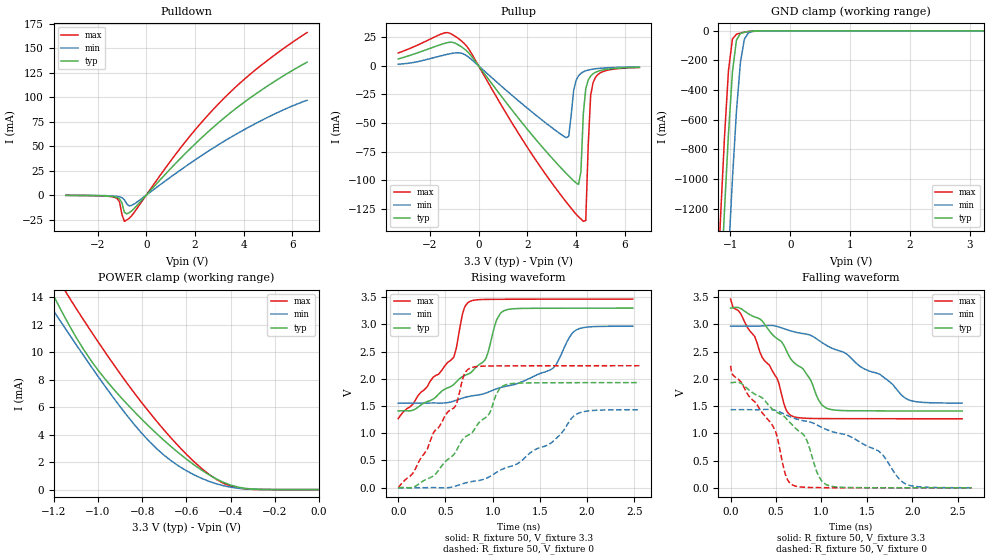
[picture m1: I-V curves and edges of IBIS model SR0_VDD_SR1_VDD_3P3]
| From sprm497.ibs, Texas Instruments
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|SR0_VSS_SR1_VSS_3P3CELL OPERATING IN SLOW MODE
|   Model Cell SR0_VDD_SR1_VDD_3P3
|SR0_VDD_SR1_VDD_3P3
[Model]   SR0_VDD_SR1_VDD_3P3
Model_type   I/O
Polarity   Non-Inverting
Enable   Active-Low
Vinl =  0.8V
Vinh =  2V
Cref =  5.0000pF
Rref =  100.0000M
Vref =  0V
Vmeas =  1.65
C_comp   2.088321p   2.017362p   2.221145p
[Model Spec]
Vinl   0.8V   0.8V   0.8V
Vinh   2V   2V   2V
[Temperature Range]   25   125   -40
[Voltage Range]   3.3   2.97   3.465
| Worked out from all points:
|   slope of the pulldown table from 0 to 0.495 V, typ, clamps not added: 36.4 ohm
|   slope of the pullup table from 0 to 0.495 V, typ, clamps not added: 34.9 ohm
|   GND clamp passes 1 mA (typ) near -0.57 V on its own axis
|   POWER clamp passes 1 mA (typ) near -0.49 V on its own axis
|   rising waveform, R_fixture 50, V_fixture 3.3: 20-80 % time 541ps typ, 710ps min, 445ps max; typ from 1.41 V to 3.3 V
|   rising waveform, R_fixture 50, V_fixture 0: 20-80 % time 550ps typ, 740ps min, 446ps max; typ from 0 V to 1.93 V
|   falling waveform, R_fixture 50, V_fixture 3.3: 20-80 % time 515ps typ, 823ps min, 401ps max; typ from 3.3 V to 1.41 V
|   falling waveform, R_fixture 50, V_fixture 0: 20-80 % time 525ps typ, 841ps min, 409ps max; typ from 1.93 V to 0.001 V
[POWER_clamp]
|   voltage   I(typ)   I(min)   I(max)
-3.3V     86.08mA    64.51mA    104.3mA
-1.267V   16.23mA    14.61mA    17.94mA
-1.233V   15.14mA    13.79mA    16.86mA
-1.2V     14.07mA    12.98mA    15.86mA
-1.133V   12.04mA    11.37mA    14.06mA
-1V       8.693mA    8.239mA    10.76mA
-866.7mV  6.192mA    5.342mA    7.695mA
-766.7mV  4.556mA    3.483mA    5.603mA
-633.3mV  2.644mA    1.698mA    3.12mA
-500mV    1.095mA    613.6uA    1.135mA
-366.7mV  181.9uA    101.9uA    111.5uA
-11.55fV  484.7nA    452.9nA    508.6nA
[Pulldown]
|   voltage   I(typ)   I(min)   I(max)
-3.3V     -240.7uA   -171.6uA   -267.5uA
-1.3V     -1.697mA   -968uA     -2.239mA
-1.1V     -3.762mA   -1.687mA   -6.636mA
-1V       -7.727mA   -2.567mA   -19.64mA
-900mV    -17.44mA   -4.637mA   -26.73mA
-800mV    -19.19mA   -8.992mA   -25.39mA
-700mV    -17.88mA   -11mA      -23.57mA
-500mV    -13.74mA   -9.146mA   -17.83mA
1.4V      37.42mA    25.57mA    48.03mA
2.9V      72.6mA     50.52mA    91.53mA
4.6V      105.1mA    74.64mA    130.4mA
6.6V      135.8mA    96.92mA    166.1mA
[Pullup]
|   voltage   I(typ)   I(min)   I(max)
-3.3V     6.015mA    1.488mA    11.26mA
-1.4V     19.63mA    9.503mA    28.79mA
-700mV    16.55mA    11.01mA    21.71mA
3.6V      -93.97mA   -62.77mA   -119mA
4.1V      -103.6mA   -8.736mA   -131.8mA
4.2V      -92.66mA   -6.55mA    -133.7mA
4.3V      -41.55mA   -5.211mA   -135.8mA
4.4V      -19.91mA   -4.314mA   -135.1mA
4.5V      -12.4mA    -3.675mA   -69.72mA
4.6V      -8.868mA   -3.197mA   -25.86mA
4.7V      -6.864mA   -2.828mA   -14.55mA
6.6V      -1.25mA    -873.6uA   -1.41mA
[GND_clamp]
|   voltage   I(typ)   I(min)   I(max)
-3.3V     -22.46A    -23.25A    -22.02A
-1.233V   -2.372A    -3.255A    -1.856A
-1.167V   -1.78A     -2.658A    -1.268A
-1.1V     -1.214A    -2.077A    -719.3mA
-1.033V   -694.8mA   -1.519A    -269mA
-966.7mV  -277.7mA   -998.2mA   -54.71mA
-900mV    -62.85mA   -543.8mA   -23.11mA
-833.3mV  -17.76mA   -212.7mA   -15.05mA
-766.7mV  -9.254mA   -55.4mA    -9.029mA
-700mV    -5.096mA   -13.88mA   -4.435mA
-633.3mV  -2.353mA   -4.844mA   -1.587mA
3.233V    464.9nA    13.45uA    453.9nA
[Ramp]
| variable   typ   min   max
dV/dt_f   1.523623/0.6823479n   1.142936/1.116097n   1.76944/0.5156569n
dV/dt_r   1.547097/0.6949547n   1.150652/0.9660429n   1.794801/0.5503525n
R_load = 50
[Rising Waveform]
R_fixture = 50
V_fixture = 3.3
V_fixture_min = 2.97
V_fixture_max = 3.465
|   time   V(typ)   V(min)   V(max)
0s        1.411V     1.554V     1.269V
588ps     1.894V     1.591V     2.394V
679ps     2.04V      1.645V     3.177V
749ps     2.094V     1.677V     3.413V
931ps     2.384V     1.74V      3.459V
1.043ns   3.086V     1.817V     3.461V
1.12ns    3.252V     1.856V     3.462V
1.638ns   3.297V     2.191V     3.464V
1.89ns    3.298V     2.902V     3.464V
2.485ns   3.299V     2.967V     3.465V
[Rising Waveform]
R_fixture = 50
V_fixture = 0
V_fixture_min = 0
V_fixture_max = 0
|   time   V(typ)   V(min)   V(max)
0s        5.618uV    6.879uV    4.844uV
154ps     4.714mV    -39.95uV   260.1mV
371ps     213.5mV    2.931mV    1.004V
616ps     679.6mV    34.54mV    1.524V
679ps     878.6mV    70.21mV    1.982V
749ps     972.5mV    103mV      2.185V
1.155ns   1.899V     375.2mV    2.238V
1.631ns   1.929V     837.2mV    2.24V
1.897ns   1.93V      1.359V     2.241V
2.555ns   1.931V     1.433V     2.241V
[Falling Waveform]
R_fixture = 50
V_fixture = 3.3
V_fixture_min = 2.97
V_fixture_max = 3.465
|   time   V(typ)   V(min)   V(max)
0s        3.3V       2.97V      3.465V
322ps     3.103V     2.97V      2.495V
511ps     2.74V      2.964V     2.012V
609ps     2.54V      2.91V      1.443V
679ps     2.333V     2.873V     1.316V
868ps     2.014V     2.808V     1.276V
1.008ns   1.515V     2.665V     1.272V
1.099ns   1.44V      2.576V     1.271V
1.96ns    1.412V     1.615V     1.269V
2.548ns   1.411V     1.557V     1.269V
[Falling Waveform]
R_fixture = 50
V_fixture = 0
V_fixture_min = 0
V_fixture_max = 0
|   time   V(typ)   V(min)   V(max)
0s        1.931V     1.436V     2.241V
469ps     1.434V     1.434V     1.124V
602ps     1.293V     1.346V     253.5mV
693ps     1.132V     1.283V     45.35mV
819ps     938.3mV    1.227V     10.77mV
966ps     226.1mV    1.142V     4.923mV
1.057ns   54.63mV    1.069V     3.752mV
1.631ns   2.688mV    674.1mV    1.147mV
1.953ns   1.576mV    53.54mV    629.5uV
2.653ns   675.9uV    3.006mV    228.5uV
